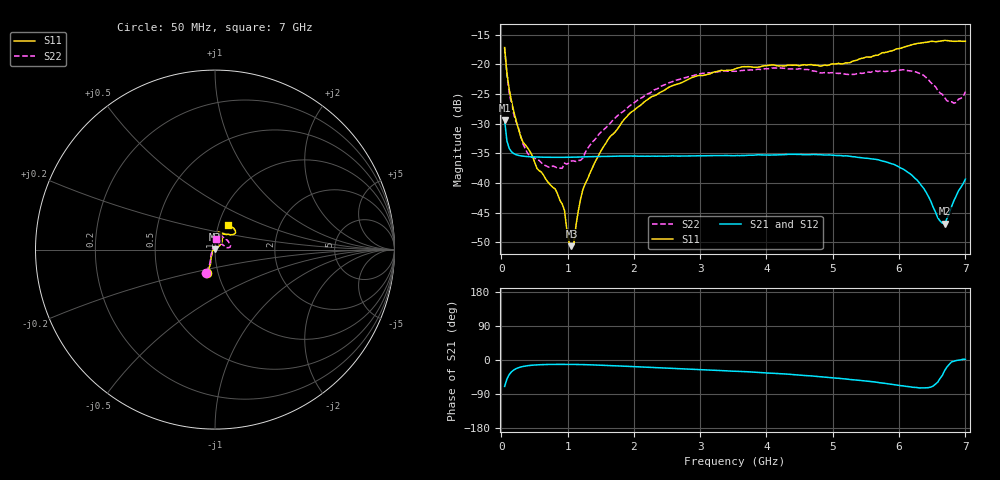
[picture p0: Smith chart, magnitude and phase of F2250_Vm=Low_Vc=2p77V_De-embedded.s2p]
! Integrated Device Technology
! Corporate Headquarters
! 6024 Silver Creek Valley Road
! San Jose, CA 95138  USA
! Phone:  1-408-284-8200
! Toll Free:  1-800-223-1366
! Webpage:  http://www.idt.com/
! Timing and RF Division
! 515 Groton Road, Suite 102
! Westford, MA 01886-6024
! Device:  F2250
! Description: Voltage Variable RF Attenuator
! Frequency:  50.0 -  6000.00 MHz
! Package:  3x3 mm Thin QFN Plastic Package: 16 pin
! Ports:  2 RF, 3 DC
!  Pin  1  = GND
!  Pin  2  = NC
!  Pin  3  = RF1  = Port 1
!  Pin  4  = NC
!  Pin  5  = GND
!  Pin  6  = GND
!  Pin  7  = GND
!  Pin  8  = GND
!  Pin  9  = NC
!  Pin 10  = RF2  = Port 2
!  Pin 11  = NC
!  Pin 12  = GND
!  Pin 13  = GND
!  Pin 14  = VCNTRL
!  Pin 15  = VDD
!  Pin 16  = VMODE
! Vcntrl:  2.770 Volts
! Vmode:  +0.000 Volts
! Vdd:  +3.30  Volts
! Current:  1.174 mA
! Data:  The device was measured on a the F2250 evaluation board which has
!  individual transmission lines to the RF pins.  Data was collected
!  using a calibrated network analyzer.  The evaluation board was
!  de-embedded using a TRL calibration technique.
!  The reference plane is the edge of the package pin.
! Misc:  SN 10
!  Action Tracker AT0258
! Date Measured:  2014-11-26
! Date:  2015-10-15  MJV
! Note:
!  Integrated Device Technology supplies this data as a sample of measured
!  data at the package pin for this product.  Your particular data for this
!  product may vary.
!  Data was taken at 25 degrees C.
!  Integrated Device Technology reserves the right to change this data at anytime.
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# GHz S dB R 50
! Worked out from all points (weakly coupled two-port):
!   201 points, 50 MHz to 7 GHz, reference 50 ohm
!   highest |S21| = -29.41 dB at 50 MHz (marker M1); lowest = -46.9 dB at 6.687 GHz (marker M2)
!   lowest |S11| = -50.7 dB at 1.058 GHz (marker M3), VSWR 1.01, Z = 49.8 + j0.242 ohm
!   |S11| at or under -10 dB: start of sweep to end of sweep
!   |S22| runs from -37.5 to -17.3 dB; largest |S21 - S12| = 6.3e-05
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0.05  -17.18 -108.7  -29.41 -69.8  -29.41 -69.8  -17.28 -111.0
0.08475  -21.45 -107.5  -32.92 -50.4  -32.92 -50.4  -21.74 -110.2
0.15425  -26.23 -116.6  -34.76 -31.1  -34.75 -31.1  -26.82 -122.4
0.29325  -32.22 -127.8  -35.43 -18.5  -35.43 -18.5  -32.09 -137.4
0.3975  -34.09 -141.9  -35.56 -15.0  -35.56 -15.0  -35.03 -160.4
0.91875  -43.53 157.8  -35.69 -11.5  -35.69 -11.5  -37.53 133.6
0.9535  -44.64 170.0  -35.68 -11.5  -35.68 -11.5  -36.65 131.2
1.023  -49.98 143.6  -35.67 -11.6  -35.67 -11.6  -36.60 116.0
1.05775  -50.65 124.1  -35.67 -11.6  -35.67 -11.6  -36.28 110.8
1.0925  -50.45 89.2  -35.65 -11.7  -35.66 -11.7  -36.29 106.3
1.162  -44.70 57.2  -35.64 -11.9  -35.64 -11.9  -36.21 95.5
1.2315  -41.09 44.5  -35.61 -12.1  -35.61 -12.1  -35.79 85.9
1.6485  -32.11 42.0  -35.52 -14.6  -35.52 -14.6  -29.88 64.6
1.96125  -28.05 42.2  -35.47 -17.2  -35.46 -17.2  -26.81 56.8
2.37825  -24.87 47.3  -35.48 -20.3  -35.48 -20.3  -23.99 56.8
3.525  -20.79 72.4  -35.40 -29.5  -35.40 -29.6  -21.19 74.7
4.7065  -20.17 72.3  -35.20 -42.5  -35.20 -42.6  -21.14 72.3
5.85325  -17.81 40.5  -36.63 -63.3  -36.63 -63.4  -21.14 23.0
6.27025  -16.51 40.0  -39.50 -72.7  -39.51 -72.7  -21.36 9.7
6.68725  -15.99 48.8  -46.86 -27.8  -46.85 -27.1  -25.64 28.6
6.861  -16.13 55.1  -42.20 -1.3  -42.14 -1.3  -26.46 57.9
7  -16.13 63.2  -39.36 1.9  -39.31 1.8  -24.62 83.1
